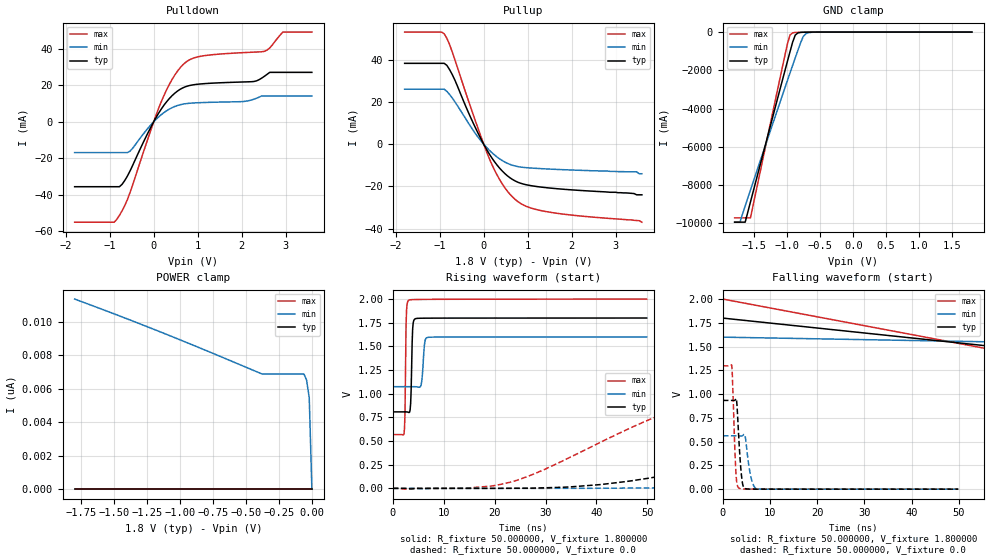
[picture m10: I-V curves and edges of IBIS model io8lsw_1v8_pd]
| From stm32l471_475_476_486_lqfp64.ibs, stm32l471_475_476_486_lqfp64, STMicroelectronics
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|   Model io8lsw_1v8_pd
[Model]  io8lsw_1v8_pd
Model_type I/O
Polarity   Non-Inverting
Enable   Active-Low
Vinl =   0.540000V
Vinh =   1.260000V
Vmeas =  0.900000V
Cref =   100.000000nF
Rref =   1.000000k
Vref =   1.800000V
C_comp   3.002600pF   2.845500pF   3.023700pF
[Temperature Range]   25.000000   0.125000k   -40.000000
[Pullup Reference]   1.800000V   1.600000V   2.000000V
[Pulldown Reference]   0.0V   0.0V   0.0V
[POWER Clamp Reference]   1.800000V   1.600000V   2.000000V
[GND Clamp Reference]   0.0V   0.0V   0.0V
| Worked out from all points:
|   slope of the pulldown table from 0 to 0.27 V, typ, clamps not added: 26.4 ohm
|   slope of the pullup table from 0 to 0.27 V, typ, clamps not added: 30.1 ohm
|   GND clamp passes 1 mA (typ) near -0.58 V on its own axis
|   rising waveform, R_fixture 50.000000, V_fixture 1.800000: 20-80 % time 262ps typ, 403ps min, 194ps max; typ from 0.808 V to 1.8 V
|   rising waveform, R_fixture 50.000000, V_fixture 0.0: 20-80 % time 64.5ns typ, 115ns min, 35.9ns max; typ from 0 V to 0.933 V
|   falling waveform, R_fixture 50.000000, V_fixture 1.800000: 20-80 % time 119ns typ, 162ns min, 92ns max; typ from 1.8 V to 0.808 V
|   falling waveform, R_fixture 50.000000, V_fixture 0.0: 20-80 % time 711ps typ, 1.02ns min, 550ps max; typ from 0.933 V to 0 V
[Pulldown]
|Voltage   I(typ)   I(min)   I(max)
-1.8V     -35.64mA   -16.93mA   -55.1mA
-840mV    -35.64mA   -16.93mA   -53.52mA
-720mV    -34.31mA   -16.93mA   -48.86mA
-540mV    -27.04mA   -16.13mA   -38.89mA
240mV     9.303mA    5.14mA     14.78mA
480mV     15.67mA    8.374mA    25.64mA
720mV     19.18mA    9.883mA    32.46mA
1.14V     20.87mA    10.54mA    36.19mA
2.28V     22.08mA    12.36mA    38.18mA
2.52V     24.95mA    14.17mA    38.63mA
2.94V     27.08mA    14.17mA    49.18mA
3.6V      27.08mA    14.17mA    49.18mA
[Pullup]
|Voltage   I(typ)   I(min)   I(max)
-1.8V     38.4mA     26.13mA    53.24mA
-900mV    38.4mA     26.13mA    52.41mA
-840mV    37.46mA    25.13mA    50.32mA
-720mV    33.23mA    22.05mA    44.01mA
-240mV    10.08mA    6.588mA    14.1mA
120mV     -4.38mA    -2.702mA   -6.45mA
420mV     -12.68mA   -7.723mA   -18.77mA
720mV     -17.48mA   -10.36mA   -26.28mA
1.02V     -19.45mA   -11.2mA    -29.89mA
1.44V     -20.65mA   -11.73mA   -32.03mA
3.48V     -24mA      -13.1mA    -36.2mA
3.6V      -24mA      -14mA      -37mA
[GND_clamp]
|Voltage   I(typ)   I(min)   I(max)
-1.8V     -9.93A     -9.932A    -9.707A
-1.72V    -9.93A     -9.932A    -9.707A
-1.64V    -9.93A     -9.083A    -9.707A
-1.56V    -8.876A    -8.251A    -9.707A
-1V       -1.54A     -2.541A    -631mA
-960mV    -1.028A    -2.139A    -153.8mA
-920mV    -527mA     -1.74A     -39.13mA
-880mV    -155.7mA   -1.344A    -18.02mA
-840mV    -45.33mA   -953mA     -12.69mA
-760mV    -8.431mA   -235mA     -7.631mA
-680mV    -3.453mA   -33.02mA   -3.876mA
1.8V      47.6uA     51.88uA    39.21uA
[POWER_clamp]
|Voltage   I(typ)   I(min)   I(max)
-1.8V     0A         11.37nA    0A
-1.14V    0A         9.374nA    0A
-380mV    0A         6.895nA    0A
-60mV     0A         6.881nA    0A
-40mV     0A         6.518nA    0A
-20mV     0A         5.452nA    0A
0V        0A         0A         0A
[Ramp]
| variable   typ   min   max
dV/dt_r  0.56008/64.46347n   0.33626/0.11513u   0.77826/35.85093n
dV/dt_f  0.59456/66.70169n   0.31128/0.11346u   0.85886/35.25965n
R_load = 50.000000
[Rising Waveform]
R_fixture= 50.000000
V_fixture= 1.800000
V_fixture_min= 1.600000
V_fixture_max= 2.000000
|time   V(typ)   V(min)   V(max)
0s        807.9mV    1.074V     568mV
2.202ns   808mV      1.074V     575.7mV
2.402ns   808mV      1.074V     804.4mV
2.703ns   807.6mV    1.074V     1.883V
3.203ns   800.9mV    1.074V     1.989V
3.504ns   892.4mV    1.074V     1.992V
3.904ns   1.684V     1.074V     1.993V
4.404ns   1.791V     1.074V     1.994V
6.807ns   1.798V     1.593V     1.996V
49.85ns   1.799V     1.599V     1.999V
[Rising Waveform]
R_fixture= 50.000000
V_fixture= 0.0
V_fixture_min= 0.0
V_fixture_max= 0.0
|time   V(typ)   V(min)   V(max)
0s        3.019nV    73.58nV    2.158nV
14.41ns   -63.81uV   -37.06uV   2.552mV
24.02ns   1.131mV    -18.48uV   79.36mV
54.05ns   143.6mV    5.762mV    806.1mV
72.07ns   334.5mV    24.97mV    1.088V
104.5ns   636mV      113.1mV    1.256V
135.7ns   800.6mV    225.6mV    1.285V
168.2ns   877.7mV    332.9mV    1.294V
259.5ns   929mV      501.1mV    1.297V
598.2ns   933.5mV    560.6mV    1.297V
[Falling Waveform]
R_fixture= 50.000000
V_fixture= 1.800000
V_fixture_min= 1.600000
V_fixture_max= 2.000000
|time   V(typ)   V(min)   V(max)
0s        1.799V     1.599V     1.999V
150.2ns   1.015V     1.467V     597.5mV
300.3ns   819.8mV    1.138V     568.6mV
450.5ns   808.8mV    1.087V     568mV
750.8ns   807.9mV    1.074V     568mV
14.86us   807.9mV    1.074V     568mV
[Falling Waveform]
R_fixture= 50.000000
V_fixture= 0.0
V_fixture_min= 0.0
V_fixture_max= 0.0
|time   V(typ)   V(min)   V(max)
0s        933.5mV    560.6mV    1.297V
1.902ns   933.5mV    560.6mV    1.304V
2.803ns   952.7mV    560.6mV    157.7mV
3.003ns   888mV      560.6mV    55.52mV
3.504ns   440.7mV    560.3mV    8.05mV
4.304ns   34.29mV    566.7mV    2.032mV
4.705ns   7.07mV     566mV      1.67mV
6.206ns   187.4uV    79.04mV    1.344mV
7.207ns   19.16uV    3.83mV     1.247mV
49.85ns   3.019nV    73.58nV    2.158nV
